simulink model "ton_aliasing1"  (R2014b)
settings: Solver=ode45  StartTime=0.0  StopTime=40.0  MaxStep=1/200  RelTol=1e-3
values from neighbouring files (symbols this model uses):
  fs = 4000    [abtast_rate_1.m]    (also in ad_test_12.m = ',     num2str(fs),'; ad_test_2.m = ',     num2str(fs),'; ad_test_3.m = ',     num2str(fs),'; DA_wandler_spektr_1.m = 100)
  tmax = 40    [ton_aliasing_1.m]    (also in ton_aliasing_2.m)
libraries: simulink x1, dspvision x1

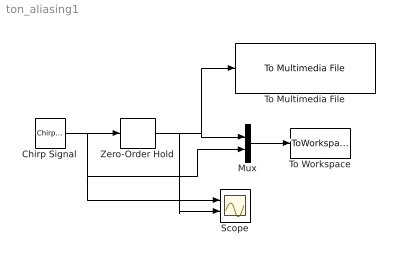
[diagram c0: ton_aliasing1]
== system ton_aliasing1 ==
  Chirp Signal : simulink/Sources/Chirp Signal  f1=0  T=tmax  f2=fmax  VectorParams1D=off
  Mux : Mux  Inputs=2
  Scope : Scope  NumInputPorts=2
  To Multimedia File : dspvision/To Multimedia File  outputFilename=audio_alias1.wav  streamSelection=Audio only  videoCompressor=None (uncompressed)  audioCompressor=None (uncompressed)  imagePorts=Separate color signals  fileType=WAV  audioDatatype=16-bit integer  fourcc=RGB  videoQuality=75  mj2000CompFactor=10
  To Workspace : ToWorkspace  VariableName=y  SaveFormat=Timeseries  SampleTime=-1
  Zero-Order Hold : ZeroOrderHold  SampleTime=1/fs
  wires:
  Zero-Order Hold/1 -> Scope/2, To Multimedia File/1, Mux/1
  Mux/1 -> To Workspace/1
  Chirp Signal/1 -> Mux/2, Scope/1, Zero-Order Hold/1
